(* Logix 5000 AddOnInstructionDefinition export EH_Liquiphant_FTL3x_IOL; software revision 38.00 *)

TYPE EH_CommAOI_Data :
STRUCT
   Device_Comm_Error : BOOL;
   CommSuccess : BOOL;
   CommFailed : BOOL;
   CommTimeOut : BOOL;
   StateDone : BOOL;
   NewState : BOOL;
   OldState : SINT;
   PortSize : SINT;
   DevicePort : SINT;
   MaxState : SINT;
   State : SINT;
   VendorID : INT;
   DeviceID : DINT;
   CyclicData : INT[16];
   AcyclicData : DINT[8];
   ReplayIndex : INT;
   AOI_Diagnostic : DINT;
   ConnectionStatus : DINT;
   OutputData : INT[16];
END_STRUCT
END_TYPE

ADD_ON_INSTRUCTION EH_Liquiphant_FTL3x_IOL   (* revision 1.0, vendor Endress+Hauser *)
// Liquiphant FTL31 Rev 1 IO-Link
// Liquiphant FTL33 Rev 1 IO-Link
VAR_IN_OUT
   DataToSend : INT[10]; {required}
   CommAOIBusy : DINT; {required}
   ActiveComPort : DINT; {required}
   DeviceAOISendRequest : DINT; {required}
   CommError : INT; {required}
   DeviceData : EH_CommAOI_Data; {required}
END_VAR
VAR_INPUT
   iExecuteRisingEdge : BOOL; {visible}
   iSetSimulation_Q1 : SINT; {visible}
   iSetSimulation_Q2 : SINT; {visible}
END_VAR
VAR_OUTPUT
   qVendor_ID : DINT; {access Read Only, visible}
   qDevice_ID : DINT; {access Read Only, visible}
   qFrequency : REAL; {visible}
   qSSO_1 : BOOL; {access Read Only, visible}
   qSimulationActiveQ1 : SINT; {visible}
   qSSO_2 : BOOL; {access Read Only, visible}
   qSimulationActiveQ2 : SINT; {access Read Only, visible}
   qAOI_Diagnostic : DINT; {access Read Only, visible}
END_VAR
VAR_IN_OUT
   qActual_Diagnostics_String : STRING; {required}
END_VAR
VAR_OUTPUT
   qActual_Diagnostics_Code : DINT; {access Read Only, visible}
END_VAR
VAR_IN_OUT
   qLast_Diagnostics_String : STRING; {required}
END_VAR
VAR_OUTPUT
   qLast_Diagnostics_Code : DINT; {access Read Only, visible}
   qCommunicationBusy : DINT; {visible}
   qCommError : INT; {access None, visible}
   qDeviceConnectionError : BOOL; {access Read Only, visible}
END_VAR
VAR_INPUT
   DeviceID1 : DINT;
   qDevice_ID_select : INT;
END_VAR
VAR
   Calc_DID : DINT; {access None}
   Calc_VID : DINT; {access None}
   Calc_Data : DINT; {access None}
   Frequency_DINT : DINT; {access None}
   Calc_Frequency : DINT; {access None}
   Calc_CondenStatus : DINT; {access None}
   CMD_Index : INT; {access None}
   CMD_Subindex : INT; {access None}
   CMD_ByteLength : INT; {access None}
   Calc_Connection_Status : DINT; {access None}
   Trigger : BOOL; {access None}
   CMD_Rd : BOOL; {access None}
   CMD_Wr : BOOL; {access None}
   Calc_Out : DINT; {access None}
   UnitSelection : REAL; {access None}
   InputByteLength : DINT;
   StateMin : DINT; {access None}
   UseDeviceUnit : BOOL; {access None}
   ActiveAOI : BOOL; {access None}
   firstTimeDone : BOOL; {access None}
   AOI_Prio : BOOL; {access None}
   TRUE : BOOL := 1; {access None}
   FALSE : BOOL; {access None}
END_VAR

ROUTINE Logic   (* structured text *)
// PMP23 Communication via AL1323
   // =======================================================================
   // Endress+Hauser Digital Solutions
   // ©Copyright (2024) All Rights Reserved
   // =======================================================================
   // Name:                EH_Liquiphant_FTL3x_IOL
   // Version:             1.0
   // Datum:               11.2025
   // Library:             01.01.00
   // Engineering:         Studio5000 V38.00.00
   // Author:              EH
   // =======================================================================
   
   
   qAOI_Diagnostic := DeviceData.AOI_Diagnostic;
   qCommunicationBusy := CommAOIBusy;
   DeviceID1 := 1024;
   StateMin := 0;
   DeviceData.MaxState := 7;
   
   if DeviceData.DevicePort = 0 or DeviceData.DeviceID <> DeviceID1 or DeviceData.ConnectionStatus <> 1 then
   
   	qVendor_ID	:= 0;
   	qDevice_ID	:= 0;
   	qFrequency	:= 0;
   	qSSO_1	:= 0;
   	qSSO_2	:= 0;
   	qSimulationActiveQ1	:= 0;
   	qActual_Diagnostics_Code	:= 0;
   	qLast_Diagnostics_Code	:= 0;
   	qLast_Diagnostics_String	:= '';
   
   	if DeviceData.DevicePort = 0 then
   
   		qActual_Diagnostics_String	:= 'Device Port is Zero';
   		DeviceData.AOI_Diagnostic.1 := TRUE;
   
   	elsif DeviceData.ConnectionStatus <> 1 then
   
   		qActual_Diagnostics_String	:= 'No Device connected';
   		qDeviceConnectionError := TRUE;
   
   	elsif DeviceData.DeviceID <> DeviceID1 then
   
   		qActual_Diagnostics_String	:= 'Wrong DeviceID';
   		DeviceData.AOI_Diagnostic.2 := TRUE;
   		qVendor_ID := DeviceData.VendorID;
   		qDevice_ID := DeviceData.DeviceID;
   
   	end_if;
   
   else
   
   	if qActual_Diagnostics_Code = 0 then
   
   		qActual_Diagnostics_String	:= '--------';
   
   	end_if;
   
   	if qLast_Diagnostics_Code = 0 then
   
   		qLast_Diagnostics_String	:= '--------';
   
   	end_if;
   
   	DeviceData.AOI_Diagnostic.1 := FALSE;
   	qDeviceConnectionError := FALSE;
   	DeviceData.AOI_Diagnostic.2  := FALSE;
   
   end_if;
   
   if not DeviceData.AOI_Diagnostic.0
   	and not qDeviceConnectionError
   	and not DeviceData.AOI_Diagnostic.2
   	and DeviceData.DevicePort > 0 or ActiveAOI and qDeviceConnectionError then
   
   
   	//*********************************
   	//Vendor ID
   	//*********************************
   
   	qVendor_ID := DeviceData.VendorID;
   
   	//*********************************
   	//Device ID
   	//*********************************
   	if DeviceData.DeviceID = DeviceID1 then
   
   		qDevice_ID_select :=1;
   
   	else
   
   		qDevice_ID_select := 0;
   
   	end_if;
   
   	qDevice_ID := DeviceData.DeviceID;
   
   	case qDevice_ID_select of  // check for Different Version
   
   	//*********************************
   	1: //FTL3x
   	//*********************************
   
   		Calc_Frequency := 0+((DeviceData.DevicePort-1)*InputByteLength);
   
   	//*********************************
   	//Process Data Frequency Liquiphant Rev 1
   	//*********************************
   
   		Frequency_DINT.0 := DeviceData.CyclicData[Calc_Frequency].0;
   		Frequency_DINT.1 := DeviceData.CyclicData[Calc_Frequency].1;
   		Frequency_DINT.2 := DeviceData.CyclicData[Calc_Frequency].2;
   		Frequency_DINT.3 := DeviceData.CyclicData[Calc_Frequency].3;
   		Frequency_DINT.4 := DeviceData.CyclicData[Calc_Frequency].4;
   		Frequency_DINT.5 := DeviceData.CyclicData[Calc_Frequency].5;
   		Frequency_DINT.6 := DeviceData.CyclicData[Calc_Frequency].6;
   		Frequency_DINT.7 := DeviceData.CyclicData[Calc_Frequency].7;
   		Frequency_DINT.8 := DeviceData.CyclicData[Calc_Frequency].8;
   		Frequency_DINT.9 := DeviceData.CyclicData[Calc_Frequency].9;
   		Frequency_DINT.10 := DeviceData.CyclicData[Calc_Frequency].10;
   		Frequency_DINT.11 := DeviceData.CyclicData[Calc_Frequency].11;
   		Frequency_DINT.12 := DeviceData.CyclicData[Calc_Frequency].12;
   		Frequency_DINT.13 := DeviceData.CyclicData[Calc_Frequency].13;
   		Frequency_DINT.14 := DeviceData.CyclicData[Calc_Frequency].13;
   		Frequency_DINT.15 := DeviceData.CyclicData[Calc_Frequency].13;
   		Frequency_DINT.16 := DeviceData.CyclicData[Calc_Frequency].13;
   		Frequency_DINT.17 := DeviceData.CyclicData[Calc_Frequency].13;
   		Frequency_DINT.18 := DeviceData.CyclicData[Calc_Frequency].13;
   		Frequency_DINT.19 := DeviceData.CyclicData[Calc_Frequency].13;
   		Frequency_DINT.20 := DeviceData.CyclicData[Calc_Frequency].13;
   		Frequency_DINT.21 := DeviceData.CyclicData[Calc_Frequency].13;
   		Frequency_DINT.22 := DeviceData.CyclicData[Calc_Frequency].13;
   		Frequency_DINT.23 := DeviceData.CyclicData[Calc_Frequency].13;
   		Frequency_DINT.24 := DeviceData.CyclicData[Calc_Frequency].13;
   		Frequency_DINT.25 := DeviceData.CyclicData[Calc_Frequency].13;
   		Frequency_DINT.26 := DeviceData.CyclicData[Calc_Frequency].13;
   		Frequency_DINT.27 := DeviceData.CyclicData[Calc_Frequency].13;
   		Frequency_DINT.28 := DeviceData.CyclicData[Calc_Frequency].13;
   		Frequency_DINT.29 := DeviceData.CyclicData[Calc_Frequency].13;
   		Frequency_DINT.30 := DeviceData.CyclicData[Calc_Frequency].13;
   		Frequency_DINT.31 := DeviceData.CyclicData[Calc_Frequency].13;
   
   
   		qFrequency := Frequency_DINT;
   
   	//*********************************
   	// Process Parameter State IO1 IO2
   	//*********************************
   
   		qSSO_1 := DeviceData.CyclicData[Calc_Frequency].14;
   		qSSO_2 := DeviceData.CyclicData[Calc_Frequency].15;
   
   		end_case;
   
   
   
   	//*********************************
   	// Checking for CommBlockBusy
   	//*********************************
   
   	if iExecuteRisingEdge and DeviceData.State = 0 then
   
   		DeviceAOISendRequest.[DeviceData.DevicePort] := 1;
   
   	end_if;
   
   
   	if ActiveComPort = DeviceData.DevicePort then
   
   		AOI_Prio :=1;
   	else
   
   		AOI_Prio := 0;
   
   	end_if;
   
   
   	if CommAOIBusy = 1 and iExecuteRisingEdge and DeviceData.State = 0 and AOI_Prio then
   
   		ActiveAOI := 1;
   
   	end_if;
   
   
   	qCommunicationBusy := CommAOIBusy;
   	qAOI_Diagnostic := DeviceData.AOI_Diagnostic;
   
   	if  ActiveAOI and qDeviceConnectionError then
   
   		DeviceData.State := DeviceData.MaxState;
   
   	end_if;
   
   
   	//*********************************
   	// State machine
   	//*********************************
   
   
   	if ActiveAOI or DeviceData.State = DeviceData.MaxState then
   
   		case DeviceData.State of
   
   		    //*********************************
   		    0: // Idle
   		    //*********************************
   
   		    // Initializing
   		   		Trigger := 0;
   			    CMD_Index := 0;
   				CMD_Subindex := 0;
   		        CMD_Wr := 0;
   				CMD_Rd := 0;
   		        CMD_ByteLength := 0;
   
   				if DeviceData.DevicePort = ActiveComPort then // check if Device is Active to reset success
   						DeviceData.CommSuccess := 0;
   						DeviceData.CommTimeOut := 0;
   						DeviceData.NewState := 1;
   						DeviceData.StateDone := 0;
   				end_if;
   
   			    // Wait for trigger
   			    if iExecuteRisingEdge and ActiveComPort = DeviceData.DevicePort then
   
   					DeviceData.AOI_Diagnostic := 0;
   					DeviceData.State := DeviceData.State + 1;
   
   			    end_if;
   
   			//*********************************
   			1: // Set Simulation Q1
   			//*********************************
   
   		        CMD_Index := 89;
   		        CMD_Subindex := 0;
   		        CMD_Wr := 1;
   				CMD_Rd := 0;
   		        CMD_ByteLength := 1;
   				DataToSend[6]:= 0;
   				DataToSend[7]:= 0;
   
   				if iSetSimulation_Q1 >= 0 and iSetSimulation_Q1 <=2 then
   
   						DataToSend[6] := iSetSimulation_Q1;
   
   						Trigger := 1;
   
   						if DeviceData.NewState then
   
   							DeviceData.StateDone := 1;
   
   						end_if;
   
   				else
   
   		            DeviceData.AOI_Diagnostic.[DeviceData.State+7] := 1;
   					DeviceData.OldState := DeviceData.State;
   			        DeviceData.State := DeviceData.State + 1;
   					DeviceData.CommSuccess := 0;
   					DeviceData.AcyclicData[0] := 0;
   					DeviceData.NewState := 1;
   
   			    end_if;
   
   				if  DeviceData.CommSuccess and DeviceData.ReplayIndex = CMD_Index then
   
   					Trigger := 0;
   					DeviceData.OldState := DeviceData.State;
   			        DeviceData.State := DeviceData.State + 1;
   					DeviceData.CommSuccess := 0;
   					DeviceData.AcyclicData[0] := 0;
   					DeviceData.NewState := 1;
   
   				 elsif DeviceData.CommTimeOut then
   
   					DeviceData.AOI_Diagnostic.[DeviceData.State+7] := 1;
   					DeviceData.OldState := DeviceData.State;
   			        DeviceData.State := DeviceData.State + 1;
   					DeviceData.CommTimeOut := 0;
   					DeviceData.AcyclicData[0] := 0;
   					DeviceData.NewState := 1;
   
   			    end_if;
   
   		    //*********************************
   		    2: // Set Simulation Q2
   		    //*********************************
   
   		        CMD_Index := 68;
   		        CMD_Subindex := 0;
   		        CMD_Wr := 1;
   				CMD_Rd := 0;
   		        CMD_ByteLength := 1;
   				DataToSend[6]:= 0;
   				DataToSend[7]:= 0;
   
   				if iSetSimulation_Q2 >= 0 and iSetSimulation_Q2 <=2 then
   
   						DataToSend[6] := iSetSimulation_Q2;
   						Trigger := 1;
   
   						if DeviceData.NewState then
   
   							DeviceData.StateDone := 1;
   
   						end_if;
   
   				else
   
   		            DeviceData.AOI_Diagnostic.[DeviceData.State+7] := 1;
   					DeviceData.OldState := DeviceData.State;
   			        DeviceData.State := DeviceData.State + 1;
   					DeviceData.CommSuccess := 0;
   					DeviceData.AcyclicData[0] := 0;
   					DeviceData.NewState := 1;
   
   			    end_if;
   
   				if  DeviceData.CommSuccess and DeviceData.ReplayIndex = CMD_Index then
   
   					Trigger := 0;
   					DeviceData.OldState := DeviceData.State;
   			        DeviceData.State := DeviceData.State + 1;
   					DeviceData.CommSuccess := 0;
   					DeviceData.AcyclicData[0] := 0;
   					DeviceData.NewState := 1;
   
   				 elsif DeviceData.CommTimeOut then
   
   					DeviceData.AOI_Diagnostic.[DeviceData.State+7] := 1;
   					DeviceData.OldState := DeviceData.State;
   			        DeviceData.State := DeviceData.State + 1;
   					DeviceData.CommTimeOut := 0;
   					DeviceData.AcyclicData[0] := 0;
   					DeviceData.NewState := 1;
   
   			    end_if;
   
   			//*********************************
   		    3: // Read Simulation Active Q1
   		    //*********************************
   
   				CMD_Index := 89;
   		        CMD_Subindex := 0;
   		        CMD_Wr := 0;
   				CMD_Rd := 1;
   		        CMD_ByteLength := 1;
   				DataToSend[6]:= 0;
   				DataToSend[7]:= 0;
   				Trigger := 1;
   				if DeviceData.NewState then
   					DeviceData.StateDone := 1;
   				end_if;
   
   				if  DeviceData.CommSuccess and DeviceData.ReplayIndex = CMD_Index then
   
   					qSimulationActiveQ1.0 := DeviceData.AcyclicData[0].0;
   					qSimulationActiveQ1.1 := DeviceData.AcyclicData[0].1;
   					qSimulationActiveQ1.2 := DeviceData.AcyclicData[0].2;
   					qSimulationActiveQ1.3 := DeviceData.AcyclicData[0].3;
   
   					Trigger := 0;
   					DeviceData.OldState := DeviceData.State;
   			        DeviceData.State := DeviceData.State + 1;
   					DeviceData.CommSuccess := 0;
   					DeviceData.AcyclicData[0] := 0;
   					DeviceData.NewState := 1;
   
   				 elsif DeviceData.CommTimeOut then
   
   					DeviceData.AOI_Diagnostic.[DeviceData.State+7] := 1;
   					DeviceData.OldState := DeviceData.State;
   			        DeviceData.State := DeviceData.State + 1;
   					DeviceData.CommTimeOut := 0;
   					DeviceData.AcyclicData[0] := 0;
   					DeviceData.NewState := 1;
   
   			    end_if;
   
   			//*********************************
   		    4: // Read Simulation Active Q2
   		    //*********************************
   
   				CMD_Index := 68;
   		        CMD_Subindex := 0;
   		        CMD_Wr := 0;
   				CMD_Rd := 1;
   		        CMD_ByteLength := 1;
   				DataToSend[6]:= 0;
   				DataToSend[7]:= 0;
   				Trigger := 1;
   
   				if DeviceData.NewState then
   
   					DeviceData.StateDone := 1;
   
   				end_if;
   
   				if  DeviceData.CommSuccess and DeviceData.ReplayIndex = CMD_Index then
   
   					qSimulationActiveQ2.0 := DeviceData.AcyclicData[0].0;
   					qSimulationActiveQ2.1 := DeviceData.AcyclicData[0].1;
   					qSimulationActiveQ2.2 := DeviceData.AcyclicData[0].2;
   					qSimulationActiveQ2.3 := DeviceData.AcyclicData[0].3;
   
   					Trigger := 0;
   					DeviceData.OldState := DeviceData.State;
   			        DeviceData.State := DeviceData.State + 1;
   					DeviceData.CommSuccess := 0;
   					DeviceData.AcyclicData[0] := 0;
   					DeviceData.NewState := 1;
   
   				 elsif DeviceData.CommTimeOut then
   
   					DeviceData.AOI_Diagnostic.[DeviceData.State+7] := 1;
   					DeviceData.OldState := DeviceData.State;
   			        DeviceData.State := DeviceData.State + 1;
   					DeviceData.CommTimeOut := 0;
   					DeviceData.AcyclicData[0] := 0;
   					DeviceData.NewState := 1;
   
   			    end_if;
   
   			//*********************************
   		    5: // Actual Diagnostic
   		    //*********************************
   
   		        CMD_Index := 260;
   		        CMD_Subindex := 0;
   		        CMD_Wr := 0;
   				CMD_Rd := 1;
   				CMD_ByteLength := 2;
   
   				Trigger := 1;
   
   				if DeviceData.NewState then
   
   					DeviceData.StateDone := 1;
   
   				end_if;
   
   				if  DeviceData.CommSuccess and DeviceData.ReplayIndex = CMD_Index then
   
   					qActual_Diagnostics_Code	:= DeviceData.AcyclicData[0];
   
   					case qActual_Diagnostics_Code of
   
   					16#2d20_2d20:
   						qActual_Diagnostics_String := 'SYSTEM OK';
   					16#0000_0001:
   						qActual_Diagnostics_String := 'no communication';
   					16#4632_3730:
   						qActual_Diagnostics_String := 'F270 - Defect in electronic / sensor';
   					16#5338_3034:
   						qActual_Diagnostics_String := 'S804 - Load current > 200mA';
   					16#4630_3432:
   						qActual_Diagnostics_String := 'F042 - Sensor corroded';
   					16#4334_3835:
   						qActual_Diagnostics_String := 'C485 - Simulation active';
   					16#4331_3832:
   						qActual_Diagnostics_String := 'C182 - Invalid calibration';
   					16#4331_3033:
   						qActual_Diagnostics_String := 'C103 - Sensor check failed';
   					16#5338_3235:
   						qActual_Diagnostics_String := 'S825 - Ambient temperature out of specification';
   					else
   						qActual_Diagnostics_String := 'Error Code unknown';
   
   			 		end_case;
   
   					Trigger := 0;
   					DeviceData.OldState := DeviceData.State;
   			        DeviceData.State := DeviceData.State + 1;
   					DeviceData.CommSuccess := 0;
   					DeviceData.AcyclicData[0] := 0;
   					DeviceData.NewState := 1;
   
   				elsif DeviceData.CommTimeOut then
   
   					DeviceData.AOI_Diagnostic.[DeviceData.State+7] := 1;
   					Trigger := 0;
   					DeviceData.OldState := DeviceData.State;
   			        DeviceData.State := DeviceData.State + 1;
   					DeviceData.CommTimeOut := 0;
   					DeviceData.AcyclicData[0] := 0;
   					DeviceData.NewState := 1;
   
   			    end_if;
   
   			//*********************************
   		    6: // Last Diagnostic
   		    //*********************************
   
   		        CMD_Index := 261;
   				CMD_Subindex := 0;
   		        CMD_Wr := 0;
   				CMD_Rd := 1;
   				CMD_ByteLength := 2;
   		        Trigger := 1;
   
   				if DeviceData.NewState then
   
   					DeviceData.StateDone := 1;
   
   				end_if;
   
   				if  DeviceData.CommSuccess and DeviceData.ReplayIndex = CMD_Index then
   
   					qLast_Diagnostics_Code := DeviceData.AcyclicData[0];
   
   					case qLast_Diagnostics_Code of
   
   					16#2D20_2D20:
   						qLast_Diagnostics_String := 'SYSTEM OK';
   					16#0000_0001:
   						qLast_Diagnostics_String := 'no communication';
   					16#4632_3730:
   						qLast_Diagnostics_String := 'F270 - Defect in electronic / sensor';
   					16#5338_3034:
   						qLast_Diagnostics_String := 'S804 - Load current > 200mA per output';
   					16#4630_3432:
   						qLast_Diagnostics_String := 'F042 - Sensor corroded';
   					16#4334_3835:
   						qLast_Diagnostics_String := 'C485 - Simulation active';
   					16#4331_3832:
   						qLast_Diagnostics_String := 'C182 - Invalid calibration';
   					16#4331_3033:
   						qLast_Diagnostics_String := 'C103 - Sensor check failed';
   					16#5338_3235:
   						qLast_Diagnostics_String := 'S825 - Ambient temperature out of specification';
   					else
   						qLast_Diagnostics_String := 'Error Code unknown';
   
   			 		end_case;
   
   					Trigger := 0;
   					DeviceData.OldState := DeviceData.State;
   			        DeviceData.State := DeviceData.State + 1;
   					DeviceData.CommSuccess := 0;
   					DeviceData.AcyclicData[0] := 0;
   					DeviceData.NewState := 1;
   
   				elsif DeviceData.CommTimeOut then
   
   					DeviceData.AOI_Diagnostic.[DeviceData.State+7] := 1;
   					Trigger := 0;
   					DeviceData.OldState := DeviceData.State;
   			        DeviceData.State := DeviceData.State + 1;
   					DeviceData.CommTimeOut := 0;
   					DeviceData.AcyclicData[0] := 0;
   					DeviceData.NewState := 1;
   
   			    end_if;
   
   			//*********************************
   		    7: // Trigger guard
   		    //*********************************
   
   				if not firstTimeDone then
   
   					CommAOIBusy := 0;
   					firstTimeDone := 1;
   					DeviceAOISendRequest.[DeviceData.DevicePort] := 0;
   					ActiveComPort := 0;
   					ActiveAOI := 0;
   					DataToSend[0] := 0;
   					DataToSend[1] := 0;
   					DataToSend[2] := 0;
   					DataToSend[3] := 0;
   					DataToSend[4] := 0;
   					DataToSend[5] := 0;
   					DataToSend[6] := 0;
   					DataToSend[7] := 0;
   					DataToSend[8] := 0;
   					DataToSend[9] := 0;
   					DeviceData.StateDone := 0;
   
   				end_if;
   
   				if DeviceData.State = DeviceData.MaxState AND NOT iExecuteRisingEdge then
   
   					DeviceData.State := 0;
   					DeviceData.OldState := DeviceData.State;
   					firstTimeDone := 0;
   
   				end_if;
   
   			end_case;
   
   		end_if;
   
   	//*************************
   	// Write Commands to the Master and the Device
   	//*************************
   	if DeviceData.State > StateMin and DeviceData.State < DeviceData.MaxState then
   
   		DataToSend[2] :=  DeviceData.DevicePort;
   		DataToSend[3] := CMD_Index;
   		DataToSend[4] := CMD_Subindex;
   		DataToSend[5].0 := CMD_Rd;
   		DataToSend[5].1 := CMD_Wr;
   		DataToSend[5].8 := CMD_ByteLength.0;
   		DataToSend[5].9 := CMD_ByteLength.1;
   		DataToSend[5].10 := CMD_ByteLength.2;
   		DataToSend[5].11 := CMD_ByteLength.3;
   		DataToSend[5].12 := CMD_ByteLength.4;
   		DataToSend[5].13 := CMD_ByteLength.5;
   		DataToSend[5].14 := CMD_ByteLength.6;
   		DataToSend[5].15 := CMD_ByteLength.7;
   
   		DataToSend[5].7 := Trigger;
   
   		qCommError	:= CommError;
   
   	end_if;
   
   end_if;
END_ROUTINE
END_ADD_ON_INSTRUCTION
